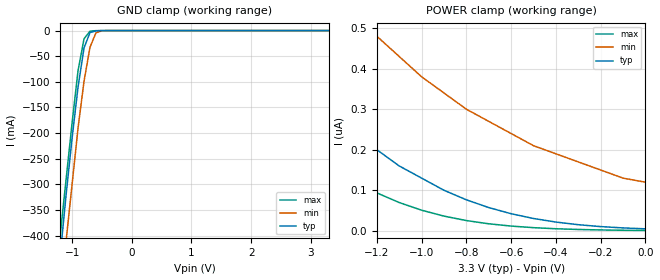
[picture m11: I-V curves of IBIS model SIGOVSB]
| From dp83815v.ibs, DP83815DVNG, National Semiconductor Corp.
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|   Model SIGOVSB
[Model]   SIGOVSB
Model_type   Input
Vinl =   0.80V
Vinh =   2.00V
Vmeas =   1.50V
Cref =  10.00pF
Rref =  50.00
C_comp   5.83pF   5.83pF   5.83pF
[Temperature Range]   27.00   100.00   0.000
[Voltage Range]   3.30V   3.00V   3.60V
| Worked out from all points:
|   GND clamp passes 1 mA (typ) near -0.61 V on its own axis
[GND_clamp]
| voltage   I(typ)   I(min)   I(max)
-3.3V     -3.09A     -3.17A     -3.06A
-1.2V     -440mA     -530mA     -400mA
-1.1V     -320mA     -410mA     -290mA
-1V       -210mA     -300mA     -180mA
-900mV    -110mA     -190mA     -77.97mA
-800mV    -33.78mA   -98.88mA   -16.01mA
-700mV    -3.91mA    -32.58mA   -1.14mA
-600mV    -530uA     -4.28mA    -130uA
-500mV    -110uA     -300uA     -10.84uA
3.3V      4.88nA     170nA      240pA
[POWER_clamp]
| voltage   I(typ)   I(min)   I(max)
-3.3V     2.26uA     2.43uA     1.98uA
-2V       700nA      1.02uA     490nA
-1.8V     550nA      860nA      360nA
-1.7V     470nA      790nA      300nA
-1.5V     350nA      660nA      200nA
-1.3V     240nA      540nA      120nA
-1.2V     200nA      480nA      93.52nA
-1V       130nA      380nA      50.84nA
-700mV    57.33nA    270nA      17.34nA
-500mV    30.41nA    210nA      7.76nA
-100mV    7.15nA     130nA      1.36nA
0V        4.88nA     120nA      870pA
